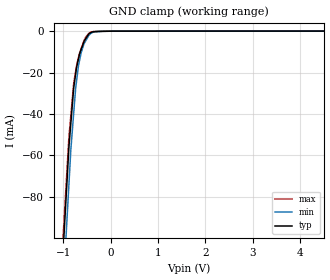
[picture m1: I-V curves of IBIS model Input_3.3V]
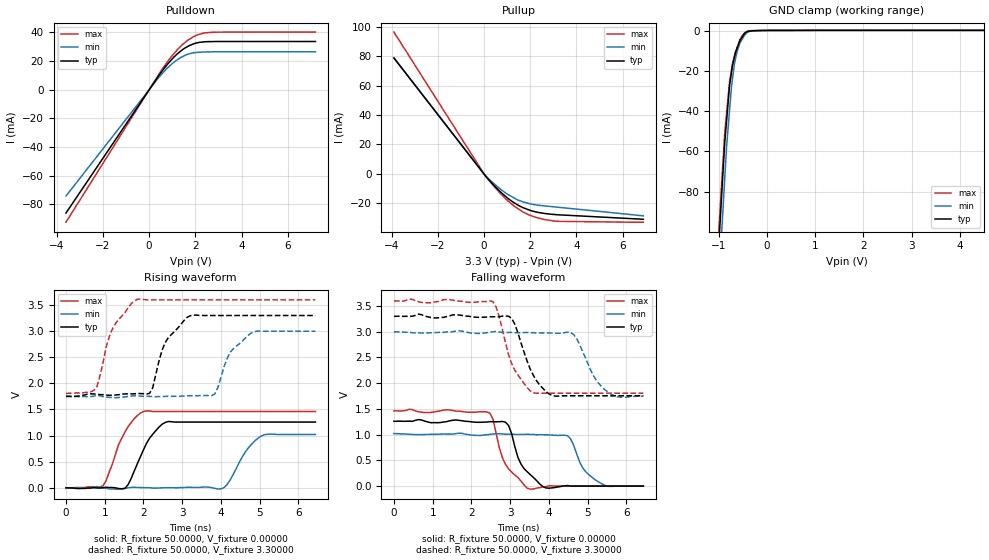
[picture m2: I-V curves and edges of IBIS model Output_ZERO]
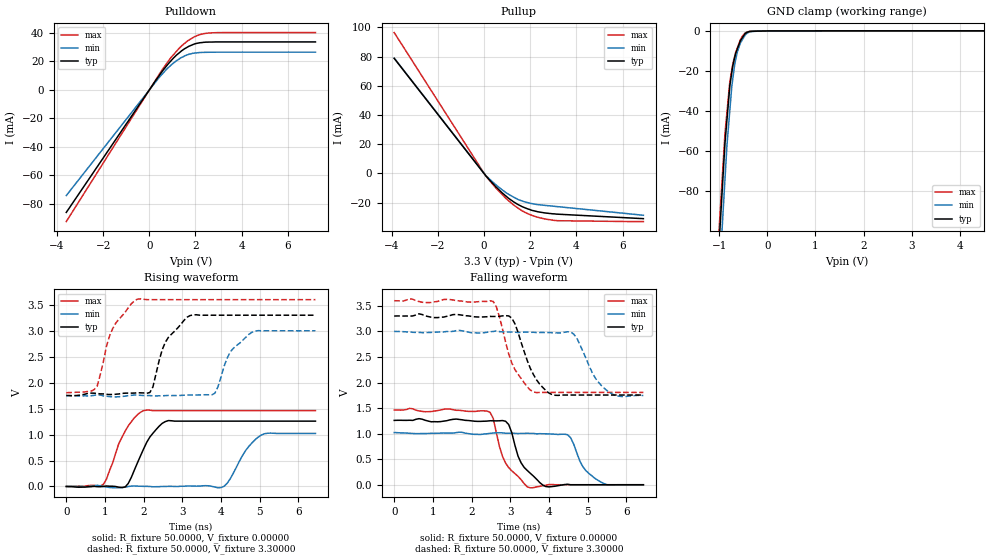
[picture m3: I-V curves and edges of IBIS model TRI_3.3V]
|Texas Instruments Incorporated
|113dB SNR 8-Channel Audio DAC with Differential Outputs
[IBIS Ver]   4.0
[Comment Char] |_char
[File Name]   pcm1791adb.ibs
[File Rev]   3.0
[Source]   Texas Instruments Incorporated.
   Analog-eLab, HPA
   12500 TI Blvd
   Dallas, TX -75243
   For Support e-mail: elab_ibis@list.ti.com
[Date]   08-17-2004
[Notes]   Quality Check of this IBIS model: Model Passes IBIS Check
   Model parses into ICX IS. Simulation done with Hyperlynx.
   1. MIN TYP MAX information is based on Temprature and Voltage
   characteristics only.
[Disclaimer]
| This model is designed as an aid for customers of Texas Instruments.
| TI and its licensors and suppliers make no warranties, either expressed
| or implied, with respect to this  model, including the warranties of
| merchantability or fitness for a particular purpose. The model is
| provided solely on an "as is" basis. The entire risk as to its quality
| and performance is with the customer.
[Copyright]
| (C) Copyright 2011 Texas Instruments Incorporated. All rights reserved.
[Component] PCM1791ADB
[Manufacturer] TI
[Package]
| variable   typ   min   max
R_pkg  1.7244E-02  1.7244E-02  1.7244E-02
L_pkg  1.8624E-09  1.8624E-09  1.8624E-09
C_pkg  5.1733E-13  5.1733E-13  5.1733E-13
[Pin] signal_name  model_name  R_pin  L_pin C_pin
1   LRCK   Input_3.3V   1.9723E-02  2.1301E-09  5.9169E-13
2   BCK   Input_3.3V   1.8868E-02  2.0377E-09  5.6604E-13
3   DATA   Input_3.3V   1.8028E-02  1.9470E-09  5.4083E-13
4   MUTE   Input_3.3V   1.7205E-02  1.8581E-09  5.1614E-13
5   SCK   Input_3.3V   1.6401E-02  1.7713E-09  4.9204E-13
6   _RST   Input_3.3V   1.5620E-02  1.6870E-09  4.6861E-13
7   VDD   POWER   1.4866E-02  1.6055E-09  4.4598E-13
8   DGND   GND   1.4866E-02  1.6055E-09  4.4598E-13
9   AGNDF   GND   1.5620E-02  1.6870E-09  4.6861E-13
10  VCCR   POWER   1.6401E-02  1.7713E-09  4.9204E-13
11  AGNDR   GND   1.7205E-02  1.8581E-09  5.1614E-13
12  VoutR-  NC   1.8028E-02  1.9470E-09  5.4083E-13
13  VoutR+  NC   1.8868E-02  2.0377E-09  5.6604E-13
14  VCOM   POWER   1.9723E-02  2.1301E-09  5.9169E-13
15  VccC   POWER   1.9723E-02  2.1301E-09  5.9169E-13
16  AGNDC   GND   1.8868E-02  2.0377E-09  5.6604E-13
17  VoutL+  NC   1.8028E-02  1.9470E-09  5.4083E-13
18  VoutL-  NC   1.7205E-02  1.8581E-09  5.1614E-13
19  AGNDL   GND   1.6401E-02  1.7713E-09  4.9204E-13
20  VccL   POWER   1.5620E-02  1.6870E-09  4.6861E-13
21  VccF   POWER   1.4866E-02  1.6055E-09  4.4598E-13
22  ZEROR   Output_ZERO  1.4866E-02  1.6055E-09  4.4598E-13
23  ZEROL   Output_ZERO  1.5620E-02  1.6870E-09  4.6861E-13
24  MSEL   Input_3.3V   1.6401E-02  1.7713E-09  4.9204E-13
25  MDO   TRI_3.3V   1.7205E-02  1.8581E-09  5.1614E-13
26  MDI   BI_3.3V   1.8028E-02  1.9470E-09  5.4083E-13
27  MC   Input_3.3V   1.8868E-02  2.0377E-09  5.6604E-13
28  _MS   BI_3.3V   1.9723E-02  2.1301E-09  5.9169E-13
| Models and submodels in the file (4): Input_3.3V (Input), Output_ZERO (Output), TRI_3.3V (3-state), BI_3.3V (I/O)
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[Model] Input_3.3V
Model_type Input
Vinl  = 800.000mV
Vinh  = 2.00000V
C_comp  2.00000pF 2.00000pF 2.00000pF
| variable   typ   min   max
[Voltage Range]   3.30000V  3.00000V  3.60000V
[POWER Clamp Reference]  3.30000V  3.00000V  3.60000V
[GND Clamp Reference]   0.00000V  0.00000V  0.00000V
[Temperature Range]   25   85   -25
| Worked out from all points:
|   GND clamp passes 1 mA (typ) near -0.45 V on its own axis
[GND Clamp]
-3.3V     -1.046A    -1.078A    -999.8mA
-881mV    -55.89mA   -73.94mA   -51.06mA
-840.9mV  -44.51mA   -57.27mA   -40.77mA
-780.3mV  -27.35mA   -39.56mA   -25.27mA
-739.7mV  -20.7mA    -27.67mA   -19.41mA
-719.4mV  -17.38mA   -23.97mA   -16.48mA
-679.1mV  -13.22mA   -16.6mA    -12.61mA
-623.4mV  -8.829mA   -10.38mA   -8.374mA
-562.1mV  -4.848mA   -6.036mA   -4.405mA
-420.8mV  -625.3uA   -1.071mA   -442.3uA
61.63mV   65.1uA     47.55uA    79.25uA
6.6V      102.1uA    79.84uA    108.8uA
[POWER Clamp]
| Voltage   I(typ)   I(min)   I(max)
-3.6V     0A         0A         0A
-3.5V     0A         0A         0A
-3.4V     0A         0A         0A
7.2V      0A         0A         0A
[Model] Output_ZERO
Model_type Output
Vref  = 0.00000V
Cref  = 2.00000pF
Vmeas = 1.65000V
C_comp  2.00000pF 2.00000pF 2.00000pF
| variable   typ   min   max
[Voltage Range]   3.30000V  3.00000V  3.60000V
[POWER Clamp Reference]  3.30000V  3.00000V  3.60000V
[Pullup Reference]   3.30000V  3.00000V  3.60000V
[Pulldown Reference]   0.00000V  0.00000V  0.00000V
[GND Clamp Reference]   0.00000V  0.00000V  0.00000V
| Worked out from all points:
|   slope of the pulldown table from 0 to 0.495 V, typ, clamps not added: 42.7 ohm
|   slope of the pullup table from 0 to 0.495 V, typ, clamps not added: 56.2 ohm
|   GND clamp passes 1 mA (typ) near -0.45 V on its own axis
|   rising waveform, R_fixture 50.0000, V_fixture 0.00000: 20-80 % time 496ps typ, 493ps min, 492ps max; typ from 0 V to 1.26 V
|   falling waveform, R_fixture 50.0000, V_fixture 0.00000: 20-80 % time 435ps typ, 434ps min, 417ps max; typ from 1.26 V to 0 V
|   falling waveform, R_fixture 50.0000, V_fixture 3.30000: 20-80 % time 473ps typ, 494ps min, 463ps max; typ from 3.3 V to 1.75 V
|   rising waveform, R_fixture 50.0000, V_fixture 3.30000: 20-80 % time 511ps typ, 508ps min, 501ps max; typ from 1.75 V to 3.3 V
[GND Clamp]
-3.3V     -1.046A    -1.078A    -999.8mA
-881mV    -55.89mA   -73.94mA   -51.06mA
-840.9mV  -44.51mA   -57.27mA   -40.77mA
-780.3mV  -27.35mA   -39.56mA   -25.27mA
-739.7mV  -20.7mA    -27.67mA   -19.41mA
-719.4mV  -17.38mA   -23.97mA   -16.48mA
-679.1mV  -13.22mA   -16.6mA    -12.61mA
-623.4mV  -8.829mA   -10.38mA   -8.374mA
-562.1mV  -4.848mA   -6.036mA   -4.405mA
-420.8mV  -625.3uA   -1.071mA   -442.3uA
61.63mV   65.1uA     47.55uA    79.25uA
6.6V      102.1uA    79.84uA    108.8uA
[Pulldown]
-3.6V     -86.06mA   -74.22mA   -92.47mA
420.6mV   9.885mA    8.601mA    10.69mA
759.5mV   17.05mA    14.64mA    18.71mA
1.042V    22.25mA    18.76mA    24.58mA
1.361V    26.87mA    22.45mA    30.24mA
1.659V    30.06mA    24.63mA    34.36mA
2.079V    32.7mA     26.03mA    38.18mA
2.579V    33.55mA    26.38mA    39.95mA
7.2V      33.64mA    26.45mA    40.2mA
[Pullup]
-3.9V     78.78mA    78.99mA    96.47mA
77.7mV    -1.836mA   -1.578mA   -1.922mA
497.8mV   -9.11mA    -7.686mA   -9.876mA
761.3mV   -13.14mA   -11.1mA    -14.23mA
1.281V    -19.61mA   -16.35mA   -21.78mA
1.661V    -22.95mA   -19.07mA   -25.85mA
1.979V    -24.84mA   -20.44mA   -28.27mA
2.358V    -26.44mA   -21.53mA   -30.25mA
3V        -27.77mA   -22.54mA   -32.2mA
6.9V      -31.07mA   -28.73mA   -33.06mA
[POWER Clamp]
| Voltage   I(typ)   I(min)   I(max)
-3.6V     0A         0A         0A
-3.5V     0A         0A         0A
-3.4V     0A         0A         0A
7.2V      0A         0A         0A
[Rising Waveform]
R_fixture = 50.0000
V_fixture = 0.00000
V_fixture_min = 0.00000
V_fixture_max = 0.00000
0s        0V         0V         0V
960ps     3.003mV    -3.257mV   42.47mV
1.52ns    -10.73mV   -13.69mV   1.064V
2ns       726.5mV    2.48mV     1.461V
2.56ns    1.251V     179.7uV    1.462V
4ns       1.259V     -20.58mV   1.462V
4.24ns    1.259V     151.6mV    1.462V
4.64ns    1.259V     697.4mV    1.462V
5.04ns    1.259V     990mV      1.462V
6.44ns    1.259V     1.022V     1.462V
[Falling Waveform]
R_fixture = 50.0000
V_fixture = 0.00000
V_fixture_min = 0.00000
V_fixture_max = 0.00000
0s        1.259V     1.022V     1.462V
2.48ns    1.252V     1.005V     1.415V
2.88ns    1.241V     1.007V     422.1mV
3.28ns    428.6mV    1.004V     98.35mV
3.52ns    222.7mV    1.003V     -60.69mV
3.92ns    -35.94mV   996.6mV    -10.98mV
4.48ns    9.761mV    978.7mV    0V
4.88ns    0V         347mV      0V
5.44ns    0V         16.16mV    0V
6.44ns    0V         0V         0V
[Falling Waveform]
R_fixture = 50.0000
V_fixture = 3.30000
V_fixture_min = 3.00000
V_fixture_max = 3.60000
0s        3.3V       3V         3.6V
2.56ns    3.291V     2.999V     3.584V
2.96ns    3.302V     2.987V     2.555V
3.12ns    3.149V     2.984V     2.254V
3.44ns    2.427V     2.986V     1.913V
3.76ns    1.969V     2.978V     1.806V
4.08ns    1.764V     2.975V     1.806V
4.56ns    1.755V     2.987V     1.806V
5.44ns    1.755V     1.879V     1.806V
6.44ns    1.755V     1.745V     1.806V
[Rising Waveform]
R_fixture = 50.0000
V_fixture = 3.30000
V_fixture_min = 3.00000
V_fixture_max = 3.60000
0s        1.755V     1.745V     1.806V
800ps     1.791V     1.767V     1.936V
1.2ns     1.772V     1.73V      3.044V
1.84ns    1.806V     1.761V     3.61V
2.16ns    1.81V      1.751V     3.6V
2.56ns    2.779V     1.751V     3.6V
3.2ns     3.294V     1.763V     3.6V
3.84ns    3.3V       1.796V     3.6V
4.8ns     3.3V       2.972V     3.6V
6.44ns    3.3V       3V         3.6V
[Ramp]
| variable  typ   min   max
dV/dt_r   755.492m/326.348p  612.017m/326.268p  874.812m/307.716p
dV/dt_f   929.998m/347.202p  754.362m/388.409p  1.07646/335.384p
R_load = 50.0000Ohms
[Model] TRI_3.3V
Model_type 3-state
Vref  = 0.00000V
Cref  = 2.00000pF
Vmeas = 1.65000V
C_comp  2.00000pF 2.00000pF 2.00000pF
| variable   typ   min   max
[Voltage Range]   3.30000V  3.00000V  3.60000V
[POWER Clamp Reference]  3.30000V  3.00000V  3.60000V
[Pullup Reference]   3.30000V  3.00000V  3.60000V
[Pulldown Reference]   0.00000V  0.00000V  0.00000V
[GND Clamp Reference]   0.00000V  0.00000V  0.00000V
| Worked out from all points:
|   slope of the pulldown table from 0 to 0.495 V, typ, clamps not added: 42.7 ohm
|   slope of the pullup table from 0 to 0.495 V, typ, clamps not added: 56.2 ohm
|   GND clamp passes 1 mA (typ) near -0.45 V on its own axis
|   rising waveform, R_fixture 50.0000, V_fixture 0.00000: 20-80 % time 496ps typ, 493ps min, 492ps max; typ from 0 V to 1.26 V
|   falling waveform, R_fixture 50.0000, V_fixture 0.00000: 20-80 % time 435ps typ, 434ps min, 417ps max; typ from 1.26 V to 0 V
|   falling waveform, R_fixture 50.0000, V_fixture 3.30000: 20-80 % time 473ps typ, 494ps min, 463ps max; typ from 3.3 V to 1.75 V
|   rising waveform, R_fixture 50.0000, V_fixture 3.30000: 20-80 % time 511ps typ, 508ps min, 501ps max; typ from 1.75 V to 3.3 V
[GND Clamp]
-3.3V     -1.046A    -1.078A    -999.8mA
-881mV    -55.89mA   -73.94mA   -51.06mA
-840.9mV  -44.51mA   -57.27mA   -40.77mA
-780.3mV  -27.35mA   -39.56mA   -25.27mA
-739.7mV  -20.7mA    -27.67mA   -19.41mA
-719.4mV  -17.38mA   -23.97mA   -16.48mA
-679.1mV  -13.22mA   -16.6mA    -12.61mA
-623.4mV  -8.829mA   -10.38mA   -8.374mA
-562.1mV  -4.848mA   -6.036mA   -4.405mA
-420.8mV  -625.3uA   -1.071mA   -442.3uA
61.63mV   65.1uA     47.55uA    79.25uA
6.6V      102.1uA    79.84uA    108.8uA
[Pulldown]
-3.6V     -86.06mA   -74.22mA   -92.47mA
420.6mV   9.885mA    8.601mA    10.69mA
759.5mV   17.05mA    14.64mA    18.71mA
1.042V    22.25mA    18.76mA    24.58mA
1.361V    26.87mA    22.45mA    30.24mA
1.659V    30.06mA    24.63mA    34.36mA
2.079V    32.7mA     26.03mA    38.18mA
2.579V    33.55mA    26.38mA    39.95mA
7.2V      33.64mA    26.45mA    40.2mA
[Pullup]
-3.9V     78.78mA    78.99mA    96.47mA
77.7mV    -1.836mA   -1.578mA   -1.922mA
497.8mV   -9.11mA    -7.686mA   -9.876mA
761.3mV   -13.14mA   -11.1mA    -14.23mA
1.281V    -19.61mA   -16.35mA   -21.78mA
1.661V    -22.95mA   -19.07mA   -25.85mA
1.979V    -24.84mA   -20.44mA   -28.27mA
2.358V    -26.44mA   -21.53mA   -30.25mA
3V        -27.77mA   -22.54mA   -32.2mA
6.9V      -31.07mA   -28.73mA   -33.06mA
[POWER Clamp]
| Voltage   I(typ)   I(min)   I(max)
-3.6V     0A         0A         0A
-3.5V     0A         0A         0A
-3.4V     0A         0A         0A
7.2V      0A         0A         0A
[Rising Waveform]
R_fixture = 50.0000
V_fixture = 0.00000
V_fixture_min = 0.00000
V_fixture_max = 0.00000
0s        0V         0V         0V
960ps     3.003mV    -3.257mV   42.47mV
1.52ns    -10.73mV   -13.69mV   1.064V
2ns       726.5mV    2.48mV     1.461V
2.56ns    1.251V     179.7uV    1.462V
4ns       1.259V     -20.58mV   1.462V
4.24ns    1.259V     151.6mV    1.462V
4.64ns    1.259V     697.4mV    1.462V
5.04ns    1.259V     990mV      1.462V
6.44ns    1.259V     1.022V     1.462V
[Falling Waveform]
R_fixture = 50.0000
V_fixture = 0.00000
V_fixture_min = 0.00000
V_fixture_max = 0.00000
0s        1.259V     1.022V     1.462V
2.48ns    1.252V     1.005V     1.415V
2.88ns    1.241V     1.007V     422.1mV
3.28ns    428.6mV    1.004V     98.35mV
3.52ns    222.7mV    1.003V     -60.69mV
3.92ns    -35.94mV   996.6mV    -10.98mV
4.48ns    9.761mV    978.7mV    0V
4.88ns    0V         347mV      0V
5.44ns    0V         16.16mV    0V
6.44ns    0V         0V         0V
[Falling Waveform]
R_fixture = 50.0000
V_fixture = 3.30000
V_fixture_min = 3.00000
V_fixture_max = 3.60000
0s        3.3V       3V         3.6V
2.56ns    3.291V     2.999V     3.584V
2.96ns    3.302V     2.987V     2.555V
3.12ns    3.149V     2.984V     2.254V
3.44ns    2.427V     2.986V     1.913V
3.76ns    1.969V     2.978V     1.806V
4.08ns    1.764V     2.975V     1.806V
4.56ns    1.755V     2.987V     1.806V
5.44ns    1.755V     1.879V     1.806V
6.44ns    1.755V     1.745V     1.806V
[Rising Waveform]
R_fixture = 50.0000
V_fixture = 3.30000
V_fixture_min = 3.00000
V_fixture_max = 3.60000
0s        1.755V     1.745V     1.806V
800ps     1.791V     1.767V     1.936V
1.2ns     1.772V     1.73V      3.044V
1.84ns    1.806V     1.761V     3.61V
2.16ns    1.81V      1.751V     3.6V
2.56ns    2.779V     1.751V     3.6V
3.2ns     3.294V     1.763V     3.6V
3.84ns    3.3V       1.796V     3.6V
4.8ns     3.3V       2.972V     3.6V
6.44ns    3.3V       3V         3.6V
[Ramp]
| variable  typ   min   max
dV/dt_r   755.492m/326.348p  612.017m/326.268p  874.812m/307.716p
dV/dt_f   929.998m/347.202p  754.362m/388.409p  1.07646/335.384p
R_load = 50.0000Ohms
